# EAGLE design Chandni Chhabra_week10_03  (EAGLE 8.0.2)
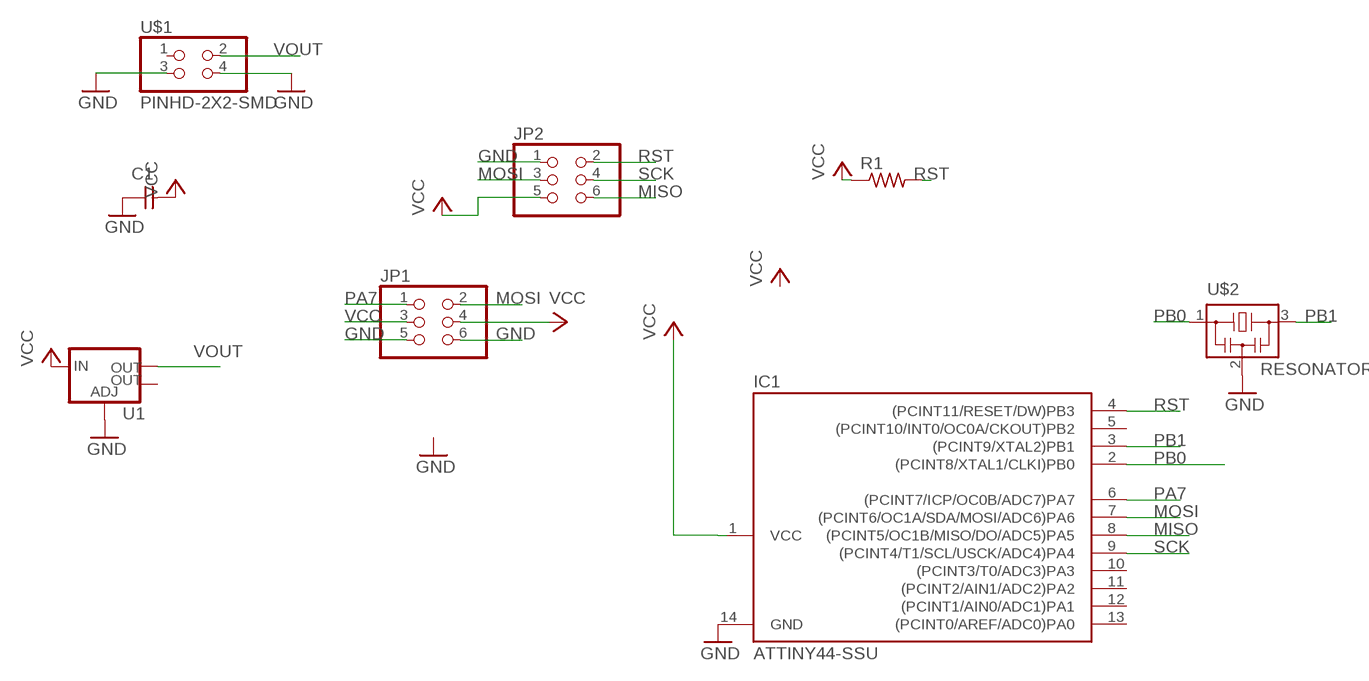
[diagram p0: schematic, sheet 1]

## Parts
C1  CAP-UNPOLARIZEDFAB  [C1206FAB]
IC1  ATTINY44-SSU  [SOIC14]
JP1  PINHD-2X3-SMD  [2X03SMD]
JP2  PINHD-2X3-SMD  [2X03SMD]
R1  RES-US1206FAB  [R1206FAB]
U1  V_REG_LM1117SOT223  [SOT223]
U$1  PINHD-2X2-SMD  [2X02SMD]
U$2  RESONATOR  [EFOBM]

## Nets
GND: C1.1 IC1.14(GND) JP1.5 JP1.6 JP2.1 U1.1(ADJ) U$1.3 U$1.4 U$2.2
MISO: IC1.8((PCINT5/OC1B/MISO/DO/ADC5)PA5) JP2.6
MOSI: IC1.7((PCINT6/OC1A/SDA/MOSI/ADC6)PA6) JP1.2 JP2.3
PA7: IC1.6((PCINT7/ICP/OC0B/ADC7)PA7) JP1.1
PB0: IC1.2((PCINT8/XTAL1/CLKI)PB0) U$2.1
PB1: IC1.3((PCINT9/XTAL2)PB1) U$2.3
RST: IC1.4((PCINT11/RESET/DW)PB3) JP2.2 R1.2
SCK: IC1.9((PCINT4/T1/SCL/USCK/ADC4)PA4) JP2.4
VCC: C1.2 IC1.1(VCC) JP1.3 JP1.4 JP2.5 R1.1 U1.3(IN)
VOUT: U1.2(OUT) U$1.2
Unconnected: IC1.5((PCINT10/INT0/OC0A/CKOUT)PB2) IC1.10((PCINT3/T0/ADC3)PA3) IC1.11((PCINT2/AIN1/ADC2)PA2) IC1.12((PCINT1/AIN0/ADC1)PA1) IC1.13((PCINT0/AREF/ADC0)PA0) U1.4(OUT) U$1.1

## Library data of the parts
C1 = fab:CAP-UNPOLARIZED
IC1 = fab:ATTINY44
JP1 JP2 = fab:PINHD-2X3-SMD: PIN HEADER
R1 = fab:RES-US: Resistor (US Symbol)
U1 = fab:V_REG_LM1117: Voltage Regulator LM1117 Standard adjustable voltage regulator but in SMD form. Spark Fun Electronics SKU : COM-00595; PROD_ID: VREG-08170
U$1 = fab:PINHD-2X2-SMD
U$2 = fab:RESONATOR

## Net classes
0 default: width 0.04 mm, clearance 0.4 mm

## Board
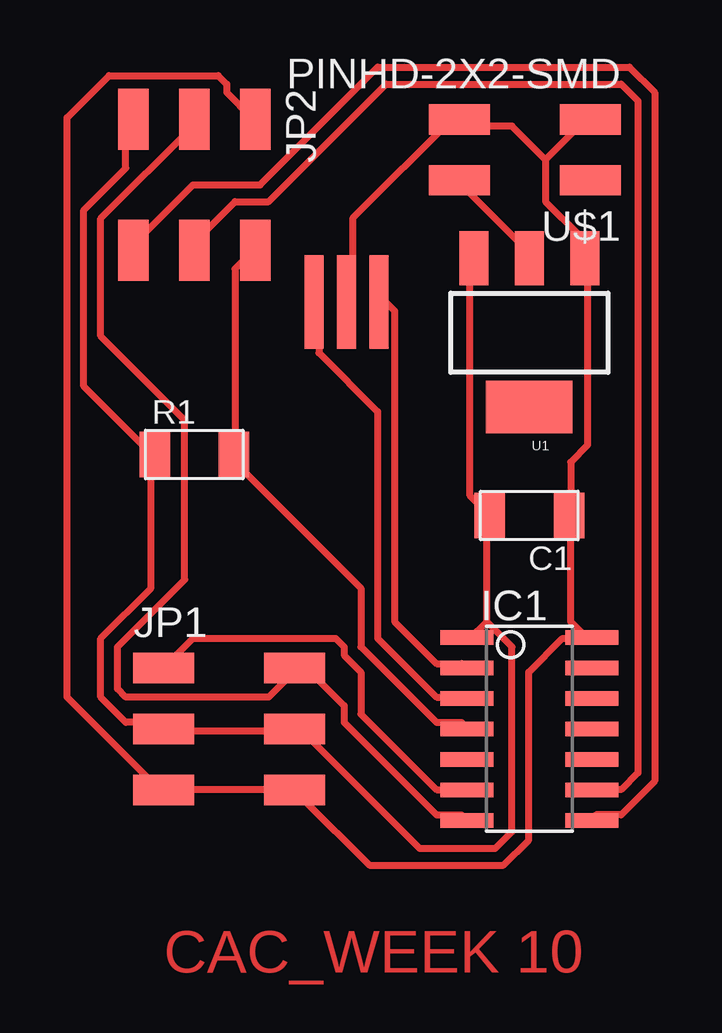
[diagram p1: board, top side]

No outline drawn. Coordinates in mm, seen from the top.
Copper layers (1*16): Top 0.035mm / dielectric 1.5mm / Bottom 0.035mm
Design rules "fab *": minimum track width 0.3mm, minimum drill 32mil, track to track 0.4mm, track to pad 0.315mm, pad to pad 0.315mm, via to via 0.315mm, smd to smd 0.315mm, copper to edge 40mil, drill to drill 16mil, minimum pad ring 10mil, minimum via ring 8mil, stop-mask expansion 4mil, vias tented up to drill 0mil, thermal gap 10mil

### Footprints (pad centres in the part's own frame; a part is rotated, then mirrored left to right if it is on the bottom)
C1206FAB = smd 1.27 x 1.905: 1 -1.651,0; 2 1.651,0
SOIC14 = smd 0.61 x 2.21: 1 -3.81,-2.603; 2 -2.54,-2.603; 3 -1.27,-2.603; 4 0,-2.603; 5 1.27,-2.603; 6 2.54,-2.603; 7 3.81,-2.603; 8 3.81,2.603; 9 2.54,2.603; 10 1.27,2.603; 11 0,2.603; 12 -1.27,2.603; 13 -2.54,2.603; 14 -3.81,2.603
2X03SMD = smd 2.54 x 1.27: 1 -2.54,2.54; 2 2.92,2.54; 3 -2.54,0; 4 2.92,0; 5 -2.54,-2.54; 6 2.92,-2.54
R1206FAB = smd 1.27 x 1.905: 1 -1.651,0; 2 1.651,0
SOT223 = smd 1.219 x 2.235: 1 -2.311,-3.099; 2 0,-3.099; 3 2.311,-3.099 | smd 3.6 x 2.2: 4 0,3.099
2X02SMD = smd 2.54 x 1.27: 1 -2.54,1.27; 2 2.92,1.27; 3 -2.54,-1.27; 4 2.92,-1.27
EFOBM = smd 0.8 x 3.9: 1 -1.35,0; 2 0,0; 3 1.35,0

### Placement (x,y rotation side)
C1  -24.13,45.72 180 top
IC1  -24.13,36.83 270 top
JP1  -36.83,36.83 0 top
JP2  -38.1,59.69 270 top
R1  -38.1,48.26 0 top
U1  -24.13,53.34 180 top
U$1  -24.13,60.96 180 top
U$2  -31.75,54.61 180 top

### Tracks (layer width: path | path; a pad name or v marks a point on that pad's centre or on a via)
GND
  Top 0.3: -21.7,40.6 -22.4,41.3 -22.4,45.5 C1.1 -22.4,45.85 -22.4,47.95 -21.7,48.65 -21.7,56.35 U1.1 -22.05,56.7 -22.05,57.4 -23.45,58.8 -23.45,60.55 | -23.45,60.55 -21.7,62.3 U$1.3 | -23.45,60.55 -24.85,61.95 -26.95,61.95 U$1.4 -27.3,62.3 -31.5,58.1 -31.5,54.95 U$2.2 | JP2.1 -35.7,62.3 -36.75,63.35 -36.75,63.7 -37.1,64.05 -41.65,64.05 -43.4,62.3 -43.4,38.15 -39.55,34.3 JP1.5 -39.2,34.3 -33.95,34.3 JP1.6 -33.6,33.95 -30.8,31.15 -25.2,31.15 -24.15,32.2 -24.15,39.2 -22.75,40.6 -21.7,40.6 | -21.7,40.6 IC1.14
MISO
  Top 0.3: IC1.8 -21.35,33.25 -20.3,33.25 -18.9,34.65 -18.9,63.35 -19.95,64.4 -30.45,64.4 -35.35,59.5 -38.15,59.5 -40.6,57.05 JP2.6
MOSI
  Top 0.3: IC1.7 -26.95,33.25 -28,33.25 -31.85,37.1 -31.85,37.8 -33.6,39.55 JP1.2 -33.95,39.2 -35,38.15 -40.95,38.15 -41.3,38.5 -41.3,40.25 -38.5,43.05 -38.5,49.7 -42,53.2 -42,58.1 -38.15,61.95 JP2.3
PA7
  Top 0.3: IC1.6 -26.95,34.3 -28,34.3 -31.15,37.45 -31.15,39.2 -31.85,39.9 -31.85,40.25 -32.2,40.6 -38.15,40.6 -39.2,39.55 JP1.1
PB0
  Top 0.3: IC1.2 -26.95,39.55 -28,39.55 -29.75,41.3 -29.75,54.25 -30.1,54.6 U$2.1
PB1
  Top 0.3: IC1.3 -26.95,38.15 -28,38.15 -30.45,40.6 -30.45,50.05 -32.9,52.5 -32.9,54.6 U$2.3
RST
  Top 0.3: JP2.2 -35.7,56.7 -36.4,56 -36.4,48.3 R1.2 -36.4,47.95 -31.15,42.7 -31.15,40.25 -28,37.1 -26.95,37.1 IC1.4
SCK
  Top 0.3: IC1.9 -21.35,34.3 -20.3,34.3 -19.6,35 -19.6,63 -20.3,63.7 -30.1,63.7 -35,58.8 -36.4,58.8 -38.15,57.05 JP2.4
VCC
  Top 0.3: -25.9,41.3 -25.9,45.5 C1.2 -25.9,45.85 -26.6,46.55 -26.6,56.35 U1.3 | -25.9,41.3 -26.6,40.6 IC1.1 | JP2.5 -40.95,61.95 -40.95,60.2 -42.7,58.45 -42.7,51.1 -39.9,48.3 R1.1 -39.9,47.95 -39.9,42.7 -42,40.6 -42,38.15 -40.95,37.1 -39.55,37.1 JP1.3 -39.2,36.75 -33.95,36.75 JP1.4 -33.6,36.75 -28.7,31.85 -25.55,31.85 -24.85,32.55 -24.85,40.25 -25.9,41.3
VOUT
  Top 0.3: U1.2 -24.15,56.7 -26.95,59.5 U$1.2

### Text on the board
Top: CAC_WEEK 10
